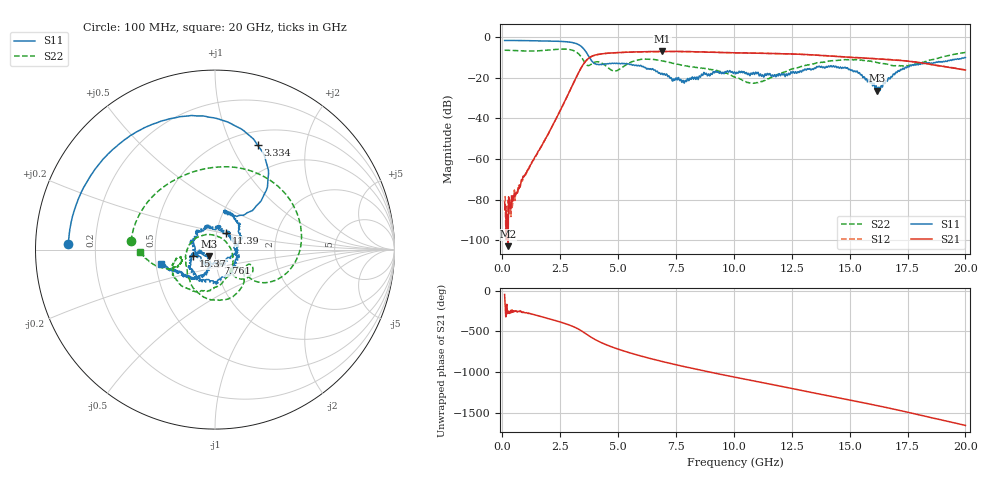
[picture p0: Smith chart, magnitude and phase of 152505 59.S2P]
!  2-Port S-parameters saved by WinCal
! VAR MeasName=S-Parameters (CALIBRATED_DATA) read from VNA (N5230C)
! VAR MeasDate=4/10/2015 9:34:45 AM
! VAR NAME=152505 59
! VAR FILENAME=152505 59.S2P
! VAR DATE=4/10/2015 9:34:45 AM
! VAR PHYS_PORTS=1,2
# Hz S DB R 50
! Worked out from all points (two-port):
!   801 points, 100 MHz to 20 GHz, reference 50 ohm
!   highest |S21| = -7.13 dB at 6.916 GHz (marker M1); lowest = -102.9 dB at 249.2 MHz (marker M2)
!   |S21| within 3 dB of the highest: 3.77 GHz to 15.13 GHz (11.36 GHz wide, 120 % of centre)
!   lowest |S11| = -26.4 dB at 16.19 GHz (marker M3), VSWR 1.10, Z = 46.7 - j3.29 ohm
!   |S11| at or under -10 dB: 3.755 GHz to end of sweep
!   |S22| runs from -22.8 to -6.0 dB; largest |S21 - S12| = 0.0063
!   S11 on the Smith chart (normalised r, x): 100 MHz: 0.10, +0.02; 3.334 GHz: 0.66, +1.26; 7.761 GHz: 1.02, -0.15; 11.39 GHz: 1.11, +0.21; 15.37 GHz: 0.78, -0.05; 20 GHz: 0.53, -0.09
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1e8  -1.75 177.6  -81.19 -45.5  -78.82 136.6  -6.56 174.3
2.4925e8  -1.75 174.1  -102.93 98.8  -80.35 100.0  -6.59 165.6
1.9905e9  -2.02 129.4  -47.59 18.4  -47.63 17.4  -6.47 73.0
2.811375e9  -2.43 99.1  -28.99 -52.0  -29.04 -52.2  -6.09 17.2
3.33375e9  -4.04 67.8  -16.71 -118.3  -16.78 -118.2  -8.78 -29.2
3.43325e9  -4.89 60.2  -14.68 -135.4  -14.72 -135.3  -10.24 -36.4
3.806375e9  -10.80 47.3  -9.88 154.7  -9.91 154.6  -13.71 -23.1
4.22925e9  -13.47 72.6  -8.45 88.8  -8.43 88.7  -12.51 -42.6
5.099875e9  -13.26 69.7  -7.62 -7.1  -7.68 -7.2  -15.60 -36.9
5.92075e9  -14.32 47.0  -7.34 -77.1  -7.37 -76.8  -11.24 -65.4
6.741625e9  -17.81 12.7  -7.17 -137.8  -7.19 -137.9  -11.47 -106.2
6.91575e9  -18.06 0.1  -7.13 -150.0  -7.19 -149.8  -11.84 -112.7
7.7615e9  -22.37 -78.8  -7.19 153.4  -7.20 153.8  -13.90 -139.9
8.80625e9  -17.87 -170.3  -7.46 88.8  -7.46 88.7  -15.59 -170.1
1.005e10  -17.50 126.1  -7.80 16.8  -7.83 16.7  -19.82 128.3
1.139325e10  -18.96 55.7  -8.11 -58.9  -8.11 -59.0  -20.99 2.7
1.338325e10  -15.70 -70.4  -8.86 -172.2  -8.83 -171.9  -13.33 -91.7
1.537325e10  -17.89 -164.3  -10.24 75.3  -10.26 75.5  -11.33 -148.5
1.619412e10  -26.40 -132.8  -10.78 26.9  -10.81 27.5  -12.63 -164.0
1.669162e10  -20.09 -105.4  -11.16 -2.8  -11.14 -3.1  -13.64 -166.8
1.801e10  -13.11 -136.0  -12.64 -87.4  -12.64 -87.1  -13.01 -155.7
2e10  -10.19 -165.4  -16.30 143.1  -16.29 143.3  -7.61 -178.3
